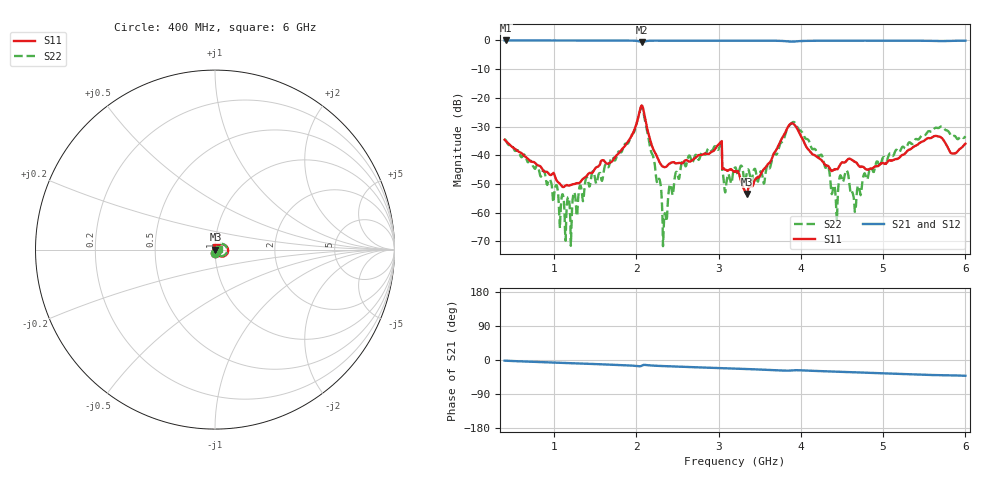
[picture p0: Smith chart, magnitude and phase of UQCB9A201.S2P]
!  Part Number  UQCB9A201	Mounting Orientation: Vertical
!  Description: RF capacitors
!  Application: Coupling, Bypass, Tuning, DC Block
!  Filters, Matching
# GHZ S DB R 50
! Freq  |S11|  S11 Ph  |S21|  S21 Ph  |S12|  S12 Ph  |S22|  S22 Ph
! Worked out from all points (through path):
!   801 points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, 400 MHz to 6 GHz, reference 50 ohm
!   highest |S21| = -0.02 dB at 421 MHz (marker M1); lowest = -0.7 dB at 2.066 GHz (marker M2)
!   group delay of S21, straight-line fit = 19.6 ps
!   lowest |S11| = -53.4 dB at 3.34 GHz (marker M3), VSWR 1.00, Z = 50.2 + j0.0199 ohm
!   |S11| at or under -10 dB: start of sweep to end of sweep
!   |S22| runs from -71.6 to -23.3 dB; largest |S21 - S12| = 0.005
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0.4  -34.59 -85.8  -0.02 -1.8  -0.01 -1.8  -34.42 -84.8
0.421  -35.20 -85.4  -0.02 -2.0  -0.01 -2.0  -35.08 -89.0
1.135  -50.63 -25.4  -0.03 -7.9  0.00 -8.0  -66.77 -65.2
1.338  -48.62 20.6  -0.04 -9.4  -0.01 -9.5  -52.63 38.0
1.856  -36.97 54.2  -0.06 -13.7  -0.03 -13.8  -36.32 76.7
2.066  -22.63 -5.4  -0.67 -15.1  -0.65 -15.2  -23.27 -4.6
2.269  -41.60 -49.6  -0.08 -15.5  -0.05 -15.6  -48.64 -66.0
2.346  -44.13 -19.2  -0.08 -16.2  -0.05 -16.3  -60.19 -10.6
2.409  -42.77 -5.4  -0.08 -16.8  -0.05 -16.9  -50.10 84.3
2.64  -42.19 17.1  -0.08 -18.6  -0.05 -18.7  -40.09 77.8
3.011  -35.86 53.7  -0.07 -21.3  -0.04 -21.4  -37.21 77.6
3.074  -44.89 -3.1  -0.07 -21.8  -0.04 -21.9  -52.12 29.4
3.2  -45.52 -11.6  -0.09 -22.8  -0.06 -22.9  -44.26 43.8
3.34  -53.42 5.3  -0.08 -23.8  -0.05 -23.9  -46.55 36.0
3.557  -44.61 47.0  -0.09 -25.6  -0.07 -25.8  -49.65 35.8
3.879  -28.94 -17.8  -0.43 -27.8  -0.41 -27.9  -29.08 -33.3
4.138  -39.56 -101.3  -0.14 -28.5  -0.12 -28.7  -37.83 -129.2
4.418  -44.80 -120.9  -0.12 -30.8  -0.11 -31.0  -52.46 -142.2
4.551  -41.98 -152.9  -0.11 -31.7  -0.10 -31.9  -45.37 -89.6
4.649  -42.21 156.1  -0.10 -32.5  -0.09 -32.6  -56.38 -164.2
5.069  -41.75 83.3  -0.09 -35.7  -0.08 -35.9  -39.91 10.7
6  -35.97 61.0  -0.09 -41.7  -0.09 -41.9  -33.36 4.2
